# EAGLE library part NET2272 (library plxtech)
NET2272 USB 2.0 Peripheral Controller Source: http://www.plxtech.com/dts/download.asp?f=NET2000/2272/Net2272.spec.re040615.pdf FBGA-Type: http://www1.plxtech.com/TEMP/77131/NET2272r1A_data_book_v1.92_31Oct05.pdf
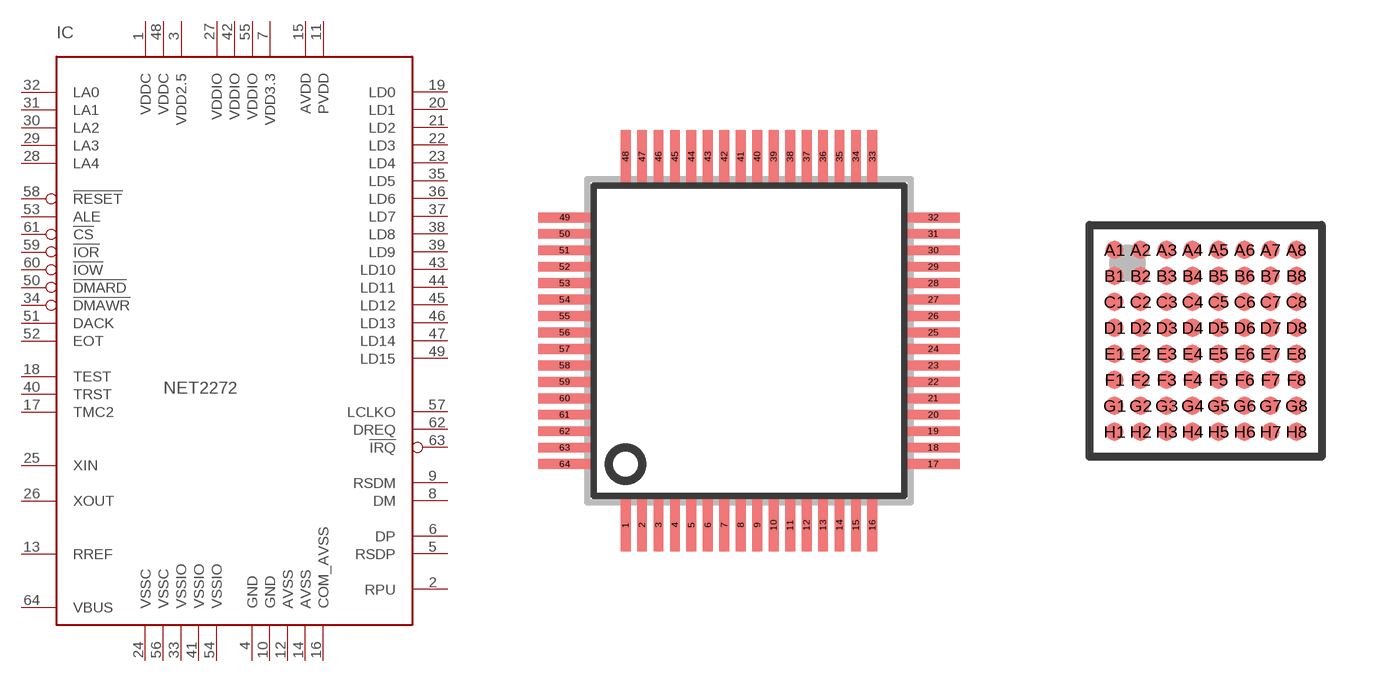
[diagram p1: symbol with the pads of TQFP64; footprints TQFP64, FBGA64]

Designator prefix IC

## NET2272REV1A-LF (MPN: NET2272REV1A-LF; OC_FARNELL: 1623121; OC_NEWARK: 08P1483)  [TQFP64]
1  VDDC  pwr
2  RPU  out
3  VDD2.5  pwr
4  GND  pwr
5  RSDP  out
6  DP
7  VDD3.3  pwr
8  DM
9  RSDM  out
10  GND  pwr
11  PVDD  pwr
12  AVSS  pwr
13  RREF  in
14  AVSS  pwr
15  AVDD  pwr
16  COM_AVSS  pwr
17  TMC2  in
18  TEST  in
19  LD0
20  LD1
21  LD2
22  LD3
23  LD4
24  VSSC  pwr
25  XIN  in
26  XOUT  out
27  VDDIO  pwr
28  LA4  in
29  LA3  in
30  LA2  in
31  LA1  in
32  LA0  in
33  VSSIO  pwr
34  !DMAWR  in
35  LD5
36  LD6
37  LD7
38  LD8
39  LD9
40  TRST  in
41  VSSIO  pwr
42  VDDIO  pwr
43  LD10
44  LD11
45  LD12
46  LD13
47  LD14
48  VDDC  pwr
49  LD15
50  !DMARD  in
51  DACK  in
52  EOT  in
53  ALE  in
54  VSSIO  pwr
55  VDDIO  pwr
56  VSSC  pwr
57  LCLKO  out
58  !RESET  in
59  !IOR  in
60  !IOW  in
61  !CS  in
62  DREQ  out
63  !IRQ  out
64  VBUS  in

## NET2272REV1A-BCF (OC_FARNELL: unknown; OC_NEWARK: unknown)  [FBGA64]
A1  LD0
A2  COM_AVSS  pwr
A3  RSDM  out
A4  GND  pwr
A5  RSDP  out
A6  GND  pwr
A7  VDDC  pwr
A8  DREQ  out
B1  LD1
B2  AVSS  pwr
B3  DM
B4  VDD3.3  pwr
B5  DP
B6  AVSS  pwr
B7  !IOW  in
B8  VBUS  in
C1  LD3
C2  LD2
C3  AVDD  pwr
C4  PVDD  pwr
C5  VDD2.5  pwr
C6  !RESET  in
C7  !CS  in
C8  !IOR  in
D1  XOUT  out
D2  VSSC  pwr
D3  LD4
D4  RREF  in
D5  RPU  out
D6  !IRQ  out
D7  VDDIO  pwr
D8  VSSC  pwr
E1  XIN  in
E2  LA3  in
E3  VDDIO  pwr
E4  TEST  in
E5  TMC2  in
E6  LCLKO  out
E7  EOT  in
E8  ALE  in
F1  LA4  in
F2  LA2  in
F3  LD7
F4  LD9
F5  VDDIO  pwr
F6  LD12
F7  DACK  in
F8  VSSIO  pwr
G1  LA0  in
G2  LA1  in
G3  LD6
G4  LD8
G5  TRST  in
G6  LD10
G7  !DMARD  in
G8  LD15
H1  VSSIO  pwr
H2  LD5
H3  !DMAWR  in
H4  VSSIO  pwr
H5  LD11
H6  LD13
H7  LD14
H8  VDDC  pwr

## Footprint TQFP64 (pad centres in mm)
64-PIN PLASTIC TQFP (10x10) shrink quad flat pack, square Source: SQFP-S-10X10-64 ipc-smd.lbr
smd 0.3 x 1.6: 1 -3.75,-5.6; 2 -3.25,-5.6; 3 -2.75,-5.6; 4 -2.25,-5.6; 5 -1.75,-5.6; 6 -1.25,-5.6; 7 -0.75,-5.6; 8 -0.25,-5.6; 9 0.25,-5.6; 10 0.75,-5.6; 11 1.25,-5.6; 12 1.75,-5.6; 13 2.25,-5.6; 14 2.75,-5.6; 15 3.25,-5.6; 16 3.75,-5.6; 33 3.75,5.6; 34 3.25,5.6; 35 2.75,5.6; 36 2.25,5.6; 37 1.75,5.6; 38 1.25,5.6; 39 0.75,5.6; 40 0.25,5.6; 41 -0.25,5.6; 42 -0.75,5.6; 43 -1.25,5.6; 44 -1.75,5.6; 45 -2.25,5.6; 46 -2.75,5.6; 47 -3.25,5.6; 48 -3.75,5.6
smd 1.6 x 0.3: 17 5.6,-3.75; 18 5.6,-3.25; 19 5.6,-2.75; 20 5.6,-2.25; 21 5.6,-1.75; 22 5.6,-1.25; 23 5.6,-0.75; 24 5.6,-0.25; 25 5.6,0.25; 26 5.6,0.75; 27 5.6,1.25; 28 5.6,1.75; 29 5.6,2.25; 30 5.6,2.75; 31 5.6,3.25; 32 5.6,3.75; 49 -5.6,3.75; 50 -5.6,3.25; 51 -5.6,2.75; 52 -5.6,2.25; 53 -5.6,1.75; 54 -5.6,1.25; 55 -5.6,0.75; 56 -5.6,0.25; 57 -5.6,-0.25; 58 -5.6,-0.75; 59 -5.6,-1.25; 60 -5.6,-1.75; 61 -5.6,-2.25; 62 -5.6,-2.75; 63 -5.6,-3.25; 64 -5.6,-3.75

## Footprint FBGA64 (pad centres in mm)
64-Ball Plastic FBGA 6 x 6 mm Source: http://www1.plxtech.com/TEMP/77131/NET2272r1A_data_book_v1.92_31Oct05.pdf
smd 0.45 x 0.45: A1 -2.275,2.275; A2 -1.625,2.275; A3 -0.975,2.275; A4 -0.325,2.275; A5 0.325,2.275; A6 0.975,2.275; A7 1.625,2.275; A8 2.275,2.275; B1 -2.275,1.625; B2 -1.625,1.625; B3 -0.975,1.625; B4 -0.325,1.625; B5 0.325,1.625; B6 0.975,1.625; B7 1.625,1.625; B8 2.275,1.625; C1 -2.275,0.975; C2 -1.625,0.975; C3 -0.975,0.975; C4 -0.325,0.975; C5 0.325,0.975; C6 0.975,0.975; C7 1.625,0.975; C8 2.275,0.975; D1 -2.275,0.325; D2 -1.625,0.325; D3 -0.975,0.325; D4 -0.325,0.325; D5 0.325,0.325; D6 0.975,0.325; D7 1.625,0.325; D8 2.275,0.325; E1 -2.275,-0.325; E2 -1.625,-0.325; E3 -0.975,-0.325; E4 -0.325,-0.325; E5 0.325,-0.325; E6 0.975,-0.325; E7 1.625,-0.325; E8 2.275,-0.325; F1 -2.275,-0.975; F2 -1.625,-0.975; F3 -0.975,-0.975; F4 -0.325,-0.975; F5 0.325,-0.975; F6 0.975,-0.975; F7 1.625,-0.975; F8 2.275,-0.975; G1 -2.275,-1.625; G2 -1.625,-1.625; G3 -0.975,-1.625; G4 -0.325,-1.625; G5 0.325,-1.625; G6 0.975,-1.625; G7 1.625,-1.625; G8 2.275,-1.625; H1 -2.275,-2.275; H2 -1.625,-2.275; H3 -0.975,-2.275; H4 -0.325,-2.275; H5 0.325,-2.275; H6 0.975,-2.275; H7 1.625,-2.275; H8 2.275,-2.275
